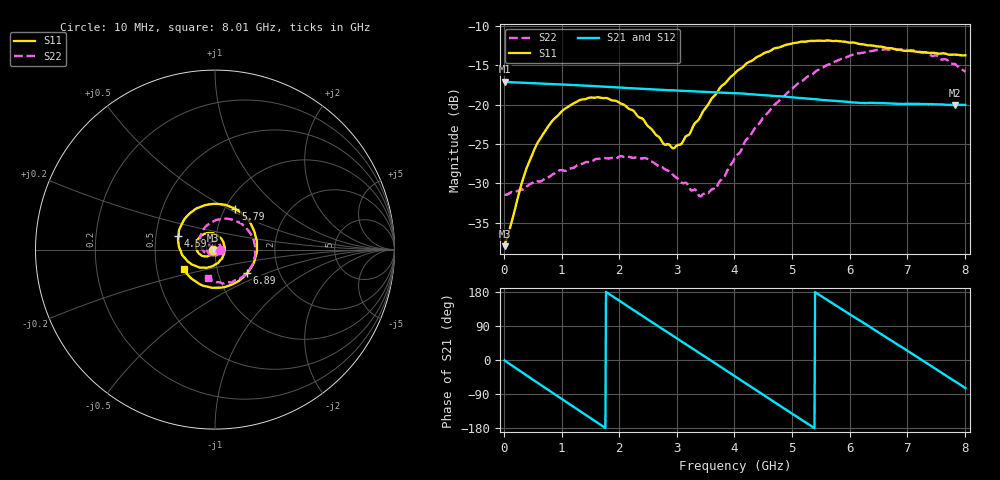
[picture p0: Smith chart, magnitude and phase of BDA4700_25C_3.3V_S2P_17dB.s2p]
!Agilent Technologies,E5071B,MY42404982,A.09.10
!Date: Mon Oct 20 18:10:10 2025
!Data & Calibration Information:
!Freq	S11:SOLT2(ON)	S21:SOLT2(ON)	S12:SOLT2(ON)	S22:SOLT2(ON)
# Hz S RI R 50
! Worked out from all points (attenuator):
!   801 points, 10 MHz to 8.01 GHz, reference 50 ohm
!   highest |S21| = -17.09 dB at 10 MHz (marker M1); lowest = -20.0 dB at 7.83 GHz (marker M2)
!   lowest |S11| = -38.0 dB at 10 MHz (marker M3), VSWR 1.03, Z = 48.8 - j0.151 ohm
!   |S11| at or under -10 dB: start of sweep to end of sweep
!   |S22| runs from -31.6 to -12.9 dB; largest |S21 - S12| = 0.0016
!   S11 on the Smith chart (normalised r, x): 10 MHz: 0.98, -0.00; 4.59 GHz: 0.66, +0.10; 5.79 GHz: 1.12, +0.54; 6.89 GHz: 1.38, -0.38; 8.01 GHz: 0.69, -0.16
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1e7  -0.0125 -0.00155  0.1398 -0.003  0.1397 -0.00313  0.0268 -0.000829
3.5e8  -0.0237 -0.0267  0.1108 -0.0816  0.1107 -0.0816  0.0227 -0.0185
5.7e8  -0.0418 -0.0376  0.0707 -0.1168  0.0705 -0.1169  0.0145 -0.0293
8.7e8  -0.0738 -0.0338  0.00137 -0.135  0.00151 -0.135  -0.00723 -0.0358
1.35e9  -0.1065 0.0166  -0.0985 -0.0885  -0.0985 -0.0885  -0.0384 -0.017
1.97e9  -0.0549 0.0891  -0.1205 0.0451  -0.1206 0.045  -0.0335 0.0315
2.45e9  0.021 0.0744  -0.0463 0.1168  -0.0465 0.1169  0.00133 0.0458
2.68e9  0.0469 0.0416  0.0025 0.1246  0.00233 0.1245  0.0179 0.0368
2.96e9  0.052 -0.0112  0.0593 0.1077  0.0593 0.1076  0.0295 0.0191
3.42e9  -0.00278 -0.0856  0.1165 0.0327  0.1167 0.0326  0.0196 -0.0174
3.68e9  -0.06 -0.1003  0.1178 -0.0209  0.1179 -0.0213  -0.000653 -0.0294
4.01e9  -0.1398 -0.0748  0.0866 -0.0807  0.0867 -0.0804  -0.0363 -0.0281
4.59e9  -0.2039 0.0739  -0.0216 -0.1123  -0.0213 -0.1126  -0.0823 0.0356
4.94e9  -0.1631 0.1788  -0.0798 -0.0783  -0.0795 -0.0789  -0.0734 0.0959
5.35e9  -0.0423 0.2502  -0.1084 -0.00752  -0.1084 -0.00831  -0.014 0.1544
5.79e9  0.1139 0.2265  -0.0822 0.0659  -0.0819 0.0661  0.0885 0.1685
6.24e9  0.2195 0.1006  -0.0149 0.1012  -0.0134 0.1016  0.1869 0.1042
6.68e9  0.2198 -0.0628  0.0577 0.0838  0.0579 0.0838  0.223 -0.0102
6.89e9  0.1798 -0.1303  0.0824 0.0584  0.0826 0.058  0.2133 -0.0706
7.34e9  0.0347 -0.2114  0.0997 -0.0149  0.0998 -0.0149  0.1344 -0.1665
7.83e9  -0.133 -0.1598  0.0554 -0.0826  0.0553 -0.0828  0.00227 -0.181
8.01e9  -0.1737 -0.1106  0.0272 -0.0959  0.0275 -0.0957  -0.0402 -0.1569
